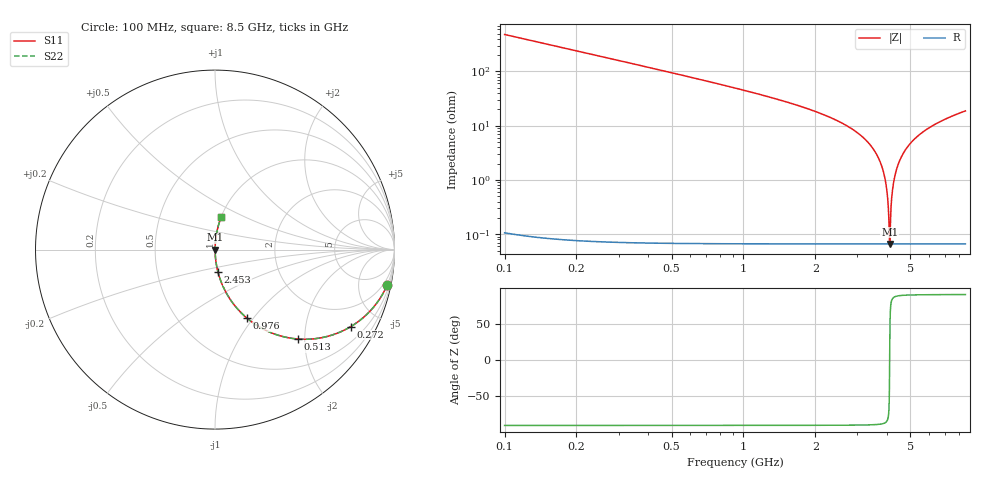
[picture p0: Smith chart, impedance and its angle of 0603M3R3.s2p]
! Created Wed Apr 18 15:34:18 2012
# hz S ma R 50
! 2 Port Network Data from SP1.SP block
! freq  magS11  angS11  magS21  angS21  magS12  angS12  magS22  angS22
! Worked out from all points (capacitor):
!   8401 points, 100 MHz to 8.5 GHz, reference 50 ohm
!   read as one part in series: C = 3.31 pF near 142 MHz
!   lowest |Z| = 66.2 mohm at 4.095 GHz (marker M1)
!   series resonance near 4.095 GHz, so ESL is about 460 pH
!   S11 on the Smith chart (normalised r, x): 100 MHz: 1.00, -9.61; 272 MHz: 1.00, -3.52; 513 MHz: 1.00, -1.85; 976 MHz: 1.00, -0.93; 2.453 GHz: 1.00, -0.25; 8.5 GHz: 1.00, +0.37
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1e8  0.979 -11.8  0.2037 78.2  0.2037 78.2  0.979 -11.8
2.72e8  0.8693 -29.6  0.4939 60.4  0.4939 60.4  0.8693 -29.6
5.13e8  0.6778 -47.3  0.7347 42.7  0.7347 42.7  0.6778 -47.3
9.76e8  0.4212 -65.0  0.9064 24.9  0.9064 24.9  0.4212 -65.0
1.5e9  0.2673 -74.4  0.963 15.5  0.963 15.5  0.2673 -74.4
2.453e9  0.1246 -82.5  0.9915 7.2  0.9915 7.2  0.1246 -82.5
2.9e9  0.08234 -84.8  0.9959 4.7  0.9959 4.7  0.08234 -84.8
3.449e9  0.04048 -86.7  0.9985 2.3  0.9985 2.3  0.04048 -86.7
3.793e9  0.01802 -86.9  0.9992 1.0  0.9992 1.0  0.01802 -86.9
3.974e9  0.007087 -84.2  0.9993 0.4  0.9993 0.4  0.007087 -84.2
4.024e9  0.004174 -80.7  0.9993 0.2  0.9993 0.2  0.004174 -80.7
4.071e9  0.001544 -64.6  0.9993 0.1  0.9993 0.1  0.001544 -64.6
4.095e9  0.0006612 -1.3  0.9993 0.0  0.9993 0.0  0.0006612 -1.3
4.121e9  0.001612 65.7  0.9993 -0.1  0.9993 -0.1  0.001612 65.7
4.16e9  0.00374 79.6  0.9993 -0.2  0.9993 -0.2  0.00374 79.6
4.194e9  0.005631 82.9  0.9993 -0.3  0.9993 -0.3  0.005631 82.9
4.3e9  0.01147 86.0  0.9993 -0.7  0.9993 -0.7  0.01147 86.0
4.489e9  0.02158 87.0  0.9991 -1.2  0.9991 -1.2  0.02158 87.0
4.772e9  0.03602 86.9  0.9987 -2.1  0.9987 -2.1  0.03602 86.9
5.7e9  0.07881 85.0  0.9962 -4.5  0.9962 -4.5  0.07881 85.0
7.1e9  0.1346 82.0  0.9902 -7.7  0.9902 -7.7  0.1346 82.0
8.5e9  0.184 79.2  0.9823 -10.6  0.9823 -10.6  0.184 79.2
